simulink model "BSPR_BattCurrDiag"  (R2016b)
settings: Solver=FixedStepDiscrete  StartTime=0.0  StopTime=10.0  FixedStep=0.02  RelTol=1e-3  EnableMultiTasking=on
undefined symbols (not defined in the file): bin2dec, BSPR_cntBattCurrDiag_CW, BSPR_cntCurrChrgDiag_CW, BSPR_cntCurrStukDiag_CW, BSPR_cntPhiCurrStuk_C, BSPR_cntVehCurrStuk_C, BSPR_cofCurrChrgFlt_C, BSPR_iCurrChrgFltThres_C, BSPR_iCurrDiagAdapThres_C, BSPR_iCurrOBCDiffThres_C, BSPR_iCurrOffsDiffThres_C, BSPR_iCurrStukDiffThres_C, BSPR_PhiCurrHiDThres_C, BSPR_PhiCurrHiUThres_C, BSPR_PhiCurrLoDThres_C, BSPR_PhiCurrLoUThres_C, BSPR_tiChrgCurrDe_C, BSPR_tiChrgCurrDiagDe_C, BSPR_tiPhiCurrDe_C, BSPR_tiVehCurrDe_C, BSPR_VehCurrHiDThres_C, BSPR_VehCurrHiUThres_C, BSPR_VehCurrLoDThres_C, BSPR_VehCurrLoUThres_C
libraries: simulink x26

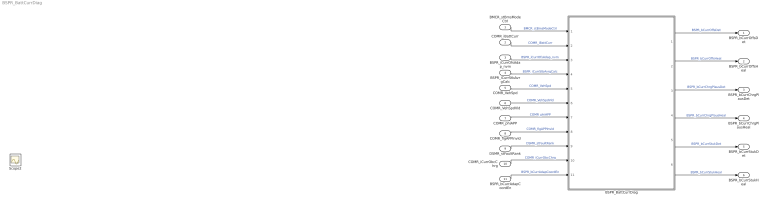
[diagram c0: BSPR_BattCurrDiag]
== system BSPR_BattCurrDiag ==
  BMCR_stBmsModeCtrl : Inport
  COMR_iBattCurr : Inport  Port=2
  BSPR_iCurrOfsAdap_nvm : Inport  Port=3
  BSPR_iCurrStbAvrgCalc : Inport  Port=4
  COMR_VehSpd : Inport  Port=5
  COMR_VehSpdVld : Inport  Port=6
  COMR_phiAPP : Inport  Port=7
  COMR_flgAPPInvld : Inport  Port=8
  DSMR_stFaultRank : Inport  Port=9
  COMR_iCurrObcChrg : Inport  Port=10
  BSPR_bCurrAdapCoordEn : Inport  Port=11
  BSPR_BattCurrDiag : Subsystem
  BSPR_bCurrOffsDet : Outport
  BSPR_bCurrOffsHeal : Outport  Port=2
  BSPR_bCurrChrgPlausDet : Outport  Port=3
  BSPR_bCurrChrgPlausHeal : Outport  Port=4
  BSPR_bCurrStukDet : Outport  Port=5
  BSPR_bCurrStukHeal : Outport  Port=6
  Scope2 : Scope
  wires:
  BMCR_stBmsModeCtrl/1 -> BSPR_BattCurrDiag/1(BMCR_stBmsModeCtrl)  "BMCR_stBmsModeCtrl"
  COMR_iBattCurr/1 -> BSPR_BattCurrDiag/2(COMR_iBattCurr)  "COMR_iBattCurr"
  BSPR_iCurrOfsAdap_nvm/1 -> BSPR_BattCurrDiag/3(BSPR_iCurrOfsAdap_nvm)  "BSPR_iCurrOfsAdap_nvm"
  COMR_iCurrObcChrg/1 -> BSPR_BattCurrDiag/10(COMR_iCurrObcChrg)  "COMR_iCurrObcChrg"
  COMR_phiAPP/1 -> BSPR_BattCurrDiag/7(COMR_phiAPP)  "COMR_phiAPP"
  COMR_VehSpd/1 -> BSPR_BattCurrDiag/5(COMR_VehSpd)  "COMR_VehSpd"
  BSPR_iCurrStbAvrgCalc/1 -> BSPR_BattCurrDiag/4(BSPR_iCurrStbAvrgCalc)  "BSPR_iCurrStbAvrgCalc"
  COMR_VehSpdVld/1 -> BSPR_BattCurrDiag/6(COMR_VehSpdVld)  "COMR_VehSpdVld"
  DSMR_stFaultRank/1 -> BSPR_BattCurrDiag/9(DSMR_stFaultRank)  "DSMR_stFaultRank"
  COMR_flgAPPInvld/1 -> BSPR_BattCurrDiag/8(COMR_flgAPPInvld)  "COMR_flgAPPInvld"
  BSPR_bCurrAdapCoordEn/1 -> BSPR_BattCurrDiag/11(BSPR_bCurrAdapCoordEn)  "BSPR_bCurrAdapCoordEn"
  BSPR_BattCurrDiag/1(BSPR_bCurrOffsDet) -> BSPR_bCurrOffsDet/1  "BSPR_bCurrOffsDet"
  BSPR_BattCurrDiag/2(BSPR_bCurrOffsHeal) -> BSPR_bCurrOffsHeal/1  "BSPR_bCurrOffsHeal"
  BSPR_BattCurrDiag/3(BSPR_bCurrChrgPlausDet) -> BSPR_bCurrChrgPlausDet/1  "BSPR_bCurrChrgPlausDet"
  BSPR_BattCurrDiag/4(BSPR_bCurrChrgPlausHeal) -> BSPR_bCurrChrgPlausHeal/1  "BSPR_bCurrChrgPlausHeal"
  BSPR_BattCurrDiag/5(BSPR_bCurrStukDet) -> BSPR_bCurrStukDet/1  "BSPR_bCurrStukDet"
  BSPR_BattCurrDiag/6(BSPR_bCurrStukHeal) -> BSPR_bCurrStukHeal/1  "BSPR_bCurrStukHeal"

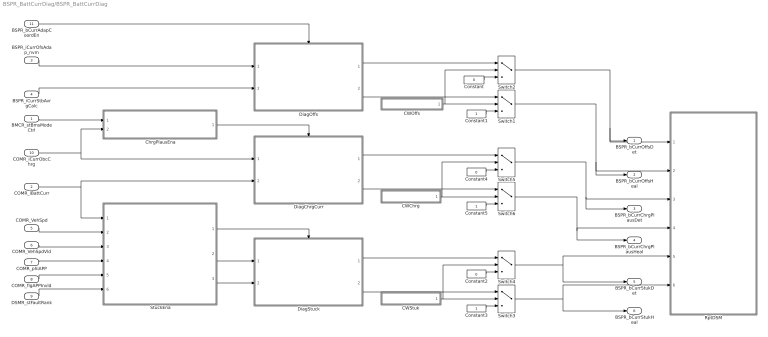
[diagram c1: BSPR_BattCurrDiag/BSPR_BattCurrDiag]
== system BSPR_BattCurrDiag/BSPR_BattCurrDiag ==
  BMCR_stBmsModeCtrl : Inport
  COMR_iBattCurr : Inport  Port=2
  BSPR_iCurrOfsAdap_nvm : Inport  Port=3
  BSPR_iCurrStbAvrgCalc : Inport  Port=4
  COMR_VehSpd : Inport  Port=5
  COMR_VehSpdVld : Inport  Port=6
  COMR_phiAPP : Inport  Port=7
  COMR_flgAPPInvld : Inport  Port=8
  DSMR_stFaultRank : Inport  Port=9
  COMR_iCurrObcChrg : Inport  Port=10
  BSPR_bCurrAdapCoordEn : Inport  Port=11
  CWChrg : Subsystem
  CWOffs : Subsystem
  CWStuk : Subsystem
  ChrgPlausEna : Subsystem  TreatAsAtomicUnit=on
  Constant : Constant  Value=0  OutDataTypeStr=boolean
  Constant1 : Constant  OutDataTypeStr=boolean
  Constant2 : Constant  Value=0  OutDataTypeStr=boolean
  Constant3 : Constant  OutDataTypeStr=boolean
  Constant4 : Constant  Value=0  OutDataTypeStr=boolean
  Constant5 : Constant  OutDataTypeStr=boolean
  DiagChrgCurr : Subsystem  TreatAsAtomicUnit=on
  DiagOffs : Subsystem
  DiagStuck : Subsystem  TreatAsAtomicUnit=on
  RptDSM : Subsystem  TreatAsAtomicUnit=on
  StuckEna : Subsystem  TreatAsAtomicUnit=on
  Switch{1..6} (6 alike) : Switch  Criteria=u2 ~= 0
  BSPR_bCurrOffsDet : Outport
  BSPR_bCurrOffsHeal : Outport  Port=2
  BSPR_bCurrChrgPlausDet : Outport  Port=3
  BSPR_bCurrChrgPlausHeal : Outport  Port=4
  BSPR_bCurrStukDet : Outport  Port=5
  BSPR_bCurrStukHeal : Outport  Port=6
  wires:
  BMCR_stBmsModeCtrl/1 -> ChrgPlausEna/1(BMCR_stBmsModeCtrl)
  BSPR_iCurrStbAvrgCalc/1 -> DiagOffs/2(BSPR_iCurrStbAvrgCalc)
  BSPR_iCurrOfsAdap_nvm/1 -> DiagOffs/1(BSPR_iCurrOfsAdap_nvm)
  StuckEna/1(BSPR_bCurrDiagStukEn) -> DiagStuck/Enable
  StuckEna/2(BSPR_iCurrMxStuk) -> DiagStuck/1(BSPR_iCurrMxStuk)
  StuckEna/3(BSPR_iCurrMnStuk) -> DiagStuck/2(BSPR_iCurrMnStuk)
  ChrgPlausEna/1(BSPR_bCurrDiagChrgPlausEn) -> DiagChrgCurr/Enable
  COMR_iCurrObcChrg/1 -> ChrgPlausEna/2(COMR_iCurrObcChrg), DiagChrgCurr/1(COMR_iCurrObcChrg)
  DSMR_stFaultRank/1 -> StuckEna/6(DSMR_stFaultRank)
  COMR_iBattCurr/1 -> StuckEna/1(COMR_iBattCurr), DiagChrgCurr/2(COMR_iBattCurr)
  COMR_flgAPPInvld/1 -> StuckEna/5(COMR_flgAPPInvld)
  COMR_phiAPP/1 -> StuckEna/4(COMR_phiAPP)
  COMR_VehSpd/1 -> StuckEna/2(COMR_VehSpd)
  COMR_VehSpdVld/1 -> StuckEna/3(COMR_VehSpdVld)
  DiagOffs/1(BSPR_bCurrOffsDet) -> Switch2/1
  Constant/1 -> Switch2/3
  CWOffs/1(~BSPR_cntBattCurrDiag_CW) -> Switch2/2, Switch1/2
  DiagOffs/2(BSPR_bCurrOffsHeal) -> Switch1/1
  Constant1/1 -> Switch1/3
  Switch2/1 -> BSPR_bCurrOffsDet/1, RptDSM/1(BSPR_bCurrOffsDet)
  Switch1/1 -> RptDSM/2(BSPR_bCurrOffsHeal), BSPR_bCurrOffsHeal/1
  CWStuk/1(BSPR_cntCurrStukDiag_CW) -> Switch4/2, Switch3/2
  DiagStuck/1(BSPR_bCurrStukDet) -> Switch4/1
  Constant2/1 -> Switch4/3
  Constant3/1 -> Switch3/3
  DiagStuck/2(BSPR_bCurrStukHeal) -> Switch3/1
  Switch4/1 -> BSPR_bCurrStukDet/1, RptDSM/5(BSPR_bCurrStukDet)
  Switch3/1 -> BSPR_bCurrStukHeal/1, RptDSM/6(BSPR_bCurrStukHeal)
  DiagChrgCurr/1(BSPR_bCurrChrgPlausDet) -> Switch5/1
  Constant4/1 -> Switch5/3
  Switch5/1 -> RptDSM/3(BSPR_bCurrChrgPlausDet), BSPR_bCurrChrgPlausDet/1
  DiagChrgCurr/2(BSPR_bCurrChrgPlausHeal) -> Switch6/1
  Constant5/1 -> Switch6/3
  CWChrg/1(BSPR_cntCurrChrgDiag_CW) -> Switch5/2, Switch6/2
  BSPR_bCurrAdapCoordEn/1 -> DiagOffs/Enable
  Switch6/1 -> BSPR_bCurrChrgPlausHeal/1, RptDSM/4(BSPR_bCurrChrgPlausHeal)

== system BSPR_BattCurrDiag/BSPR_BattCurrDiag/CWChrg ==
  Bitwise Operator : simulink/Logic and Bit Operations/Bitwise Operator  logicop=AND  UseBitMask=on  BitMask=bin2dec('00000001')  BitMaskRealWorld=Stored Integer
  Compare To Constant : simulink/Logic and Bit Operations/Compare To Constant  relop===  const=1  OutDataTypeStr=boolean
  Constant7 : Constant  Value=BSPR_cntCurrChrgDiag_CW
  BSPR_cntCurrChrgDiag_CW : Outport
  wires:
  Constant7/1 -> Bitwise Operator/1
  Bitwise Operator/1 -> Compare To Constant/1
  Compare To Constant/1 -> BSPR_cntCurrChrgDiag_CW/1

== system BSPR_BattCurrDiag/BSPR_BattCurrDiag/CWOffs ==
  Bitwise Operator : simulink/Logic and Bit Operations/Bitwise Operator  logicop=AND  UseBitMask=on  BitMask=bin2dec('00000001')  BitMaskRealWorld=Stored Integer
  Compare To Constant : simulink/Logic and Bit Operations/Compare To Constant  relop===  const=1  OutDataTypeStr=boolean
  Constant7 : Constant  Value=BSPR_cntBattCurrDiag_CW
  ~BSPR_cntBattCurrDiag_CW : Outport
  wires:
  Constant7/1 -> Bitwise Operator/1
  Bitwise Operator/1 -> Compare To Constant/1
  Compare To Constant/1 -> ~BSPR_cntBattCurrDiag_CW/1

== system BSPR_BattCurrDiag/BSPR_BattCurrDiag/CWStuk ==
  Bitwise Operator : simulink/Logic and Bit Operations/Bitwise Operator  logicop=AND  UseBitMask=on  BitMask=bin2dec('00000001')  BitMaskRealWorld=Stored Integer
  Compare To Constant : simulink/Logic and Bit Operations/Compare To Constant  relop===  const=1  OutDataTypeStr=boolean
  Constant7 : Constant  Value=BSPR_cntCurrStukDiag_CW
  BSPR_cntCurrStukDiag_CW : Outport
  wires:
  Compare To Constant/1 -> BSPR_cntCurrStukDiag_CW/1
  Bitwise Operator/1 -> Compare To Constant/1
  Constant7/1 -> Bitwise Operator/1

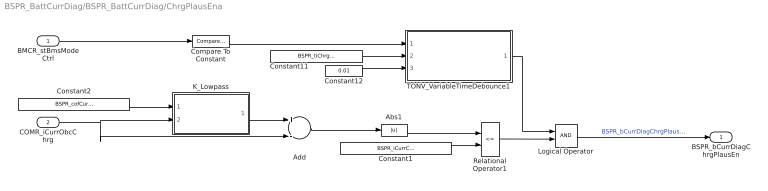
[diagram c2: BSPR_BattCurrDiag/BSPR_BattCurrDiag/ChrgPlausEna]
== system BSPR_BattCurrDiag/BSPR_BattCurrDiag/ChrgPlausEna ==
  BMCR_stBmsModeCtrl : Inport
  COMR_iCurrObcChrg : Inport  Port=2
  Abs1 : Abs
  Add : Sum  Inputs=+-
  Compare To Constant : simulink/Logic and Bit Operations/Compare To Constant  relop===  const=6  OutDataTypeStr=boolean
  Constant1 : Constant  Value=BSPR_iCurrChrgFltThres_C
  Constant11 : Constant  Value=BSPR_tiChrgCurrDe_C
  Constant12 : Constant  Value=0.01
  Constant2 : Constant  Value=BSPR_cofCurrChrgFlt_C
  K_Lowpass : Subsystem  TreatAsAtomicUnit=on  RTWFcnName=K_Lowpass  RTWFileName=SrvLib
  Logical Operator : Logic  AllPortsSameDT=off  OutDataTypeStr=boolean
  Relational Operator1 : RelationalOperator  Operator=<=  OutDataTypeStr=boolean  RndMeth=Simplest
  TONV_VariableTimeDebounce1 : Subsystem  TreatAsAtomicUnit=on  RTWFcnName=TONV_VariableTimeDebounce  RTWFileName=SrvLib
  BSPR_bCurrDiagChrgPlausEn : Outport
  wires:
  BMCR_stBmsModeCtrl/1 -> Compare To Constant/1
  Constant11/1 -> TONV_VariableTimeDebounce1/2(T)
  Constant12/1 -> TONV_VariableTimeDebounce1/3(dT)
  Compare To Constant/1 -> TONV_VariableTimeDebounce1/1(u)
  TONV_VariableTimeDebounce1/1(y) -> Logical Operator/1
  Constant1/1 -> Relational Operator1/2
  Abs1/1 -> Relational Operator1/1
  COMR_iCurrObcChrg/1 -> Add/2, K_Lowpass/2(u)
  Constant2/1 -> K_Lowpass/1(k)
  K_Lowpass/1(y) -> Add/1
  Add/1 -> Abs1/1
  Relational Operator1/1 -> Logical Operator/2
  Logical Operator/1 -> BSPR_bCurrDiagChrgPlausEn/1  "BSPR_bCurrDiagChrgPlausEn"

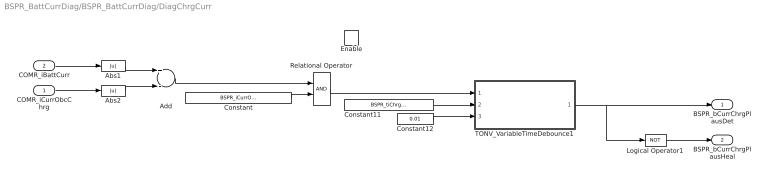
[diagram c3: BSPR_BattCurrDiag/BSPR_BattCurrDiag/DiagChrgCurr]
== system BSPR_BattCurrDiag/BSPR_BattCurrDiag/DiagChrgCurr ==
  COMR_iCurrObcChrg : Inport
  COMR_iBattCurr : Inport  Port=2
  Enable : EnablePort
  Abs1 : Abs
  Abs2 : Abs
  Add : Sum  Inputs=+-
  Constant : Constant  Value=BSPR_iCurrOBCDiffThres_C
  Constant11 : Constant  Value=BSPR_tiChrgCurrDiagDe_C
  Constant12 : Constant  Value=0.01
  Logical Operator1 : Logic  Operator=NOT  Inputs=1  AllPortsSameDT=off  OutDataTypeStr=boolean
  Relational Operator : RelationalOperator  OutDataTypeStr=boolean  RndMeth=Simplest
  TONV_VariableTimeDebounce1 : Subsystem  TreatAsAtomicUnit=on  RTWFcnName=TONV_VariableTimeDebounce  RTWFileName=SrvLib
  BSPR_bCurrChrgPlausDet : Outport
  BSPR_bCurrChrgPlausHeal : Outport  Port=2
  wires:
  COMR_iBattCurr/1 -> Abs1/1
  Constant/1 -> Relational Operator/2
  Logical Operator1/1 -> BSPR_bCurrChrgPlausHeal/1
  Constant11/1 -> TONV_VariableTimeDebounce1/2(T)
  Constant12/1 -> TONV_VariableTimeDebounce1/3(dT)
  Relational Operator/1 -> TONV_VariableTimeDebounce1/1(u)
  TONV_VariableTimeDebounce1/1(y) -> BSPR_bCurrChrgPlausDet/1, Logical Operator1/1
  Abs1/1 -> Add/1
  COMR_iCurrObcChrg/1 -> Abs2/1
  Add/1 -> Relational Operator/1
  Abs2/1 -> Add/2

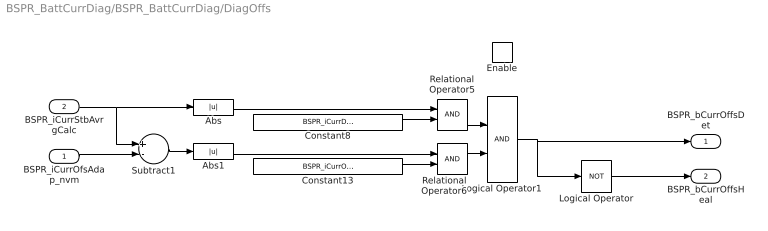
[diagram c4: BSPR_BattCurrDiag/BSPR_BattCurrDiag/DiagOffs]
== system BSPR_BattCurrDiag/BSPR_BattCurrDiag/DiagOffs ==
  BSPR_iCurrOfsAdap_nvm : Inport
  BSPR_iCurrStbAvrgCalc : Inport  Port=2
  Enable : EnablePort  StatesWhenEnabling=reset  PropagateVarSize=During execution  ZeroCross=off
  Abs : Abs
  Abs1 : Abs
  Constant13 : Constant  Value=BSPR_iCurrOffsDiffThres_C  OutDataTypeStr=single
  Constant8 : Constant  Value=BSPR_iCurrDiagAdapThres_C  OutDataTypeStr=single
  Logical Operator : Logic  Operator=NOT  Inputs=1  AllPortsSameDT=off  OutDataTypeStr=boolean
  Logical Operator1 : Logic  AllPortsSameDT=off  OutDataTypeStr=boolean
  Relational Operator5 : RelationalOperator  OutDataTypeStr=boolean  RndMeth=Simplest
  Relational Operator6 : RelationalOperator  OutDataTypeStr=boolean  RndMeth=Simplest
  Subtract1 : Sum  Inputs=+-
  BSPR_bCurrOffsDet : Outport
  BSPR_bCurrOffsHeal : Outport  Port=2
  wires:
  Constant8/1 -> Relational Operator5/2
  Constant13/1 -> Relational Operator6/2
  Logical Operator1/1 -> BSPR_bCurrOffsDet/1, Logical Operator/1
  BSPR_iCurrStbAvrgCalc/1 -> Subtract1/1, Abs/1
  Abs/1 -> Relational Operator5/1
  Subtract1/1 -> Abs1/1
  Abs1/1 -> Relational Operator6/1
  BSPR_iCurrOfsAdap_nvm/1 -> Subtract1/2
  Relational Operator5/1 -> Logical Operator1/1
  Relational Operator6/1 -> Logical Operator1/2
  Logical Operator/1 -> BSPR_bCurrOffsHeal/1

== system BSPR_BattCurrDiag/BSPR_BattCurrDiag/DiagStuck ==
  BSPR_iCurrMxStuk : Inport
  BSPR_iCurrMnStuk : Inport  Port=2
  Enable : EnablePort
  Add : Sum  Inputs=+-
  Constant : Constant  Value=BSPR_iCurrStukDiffThres_C
  Logical Operator : Logic  Operator=NOT  Inputs=1  AllPortsSameDT=off  OutDataTypeStr=boolean
  Relational Operator : RelationalOperator  Operator=<=  OutDataTypeStr=boolean  RndMeth=Simplest
  BSPR_bCurrStukDet : Outport
  BSPR_bCurrStukHeal : Outport  Port=2
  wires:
  Add/1 -> Relational Operator/1
  Constant/1 -> Relational Operator/2
  Relational Operator/1 -> Logical Operator/1, BSPR_bCurrStukDet/1
  BSPR_iCurrMxStuk/1 -> Add/1
  BSPR_iCurrMnStuk/1 -> Add/2
  Logical Operator/1 -> BSPR_bCurrStukHeal/1

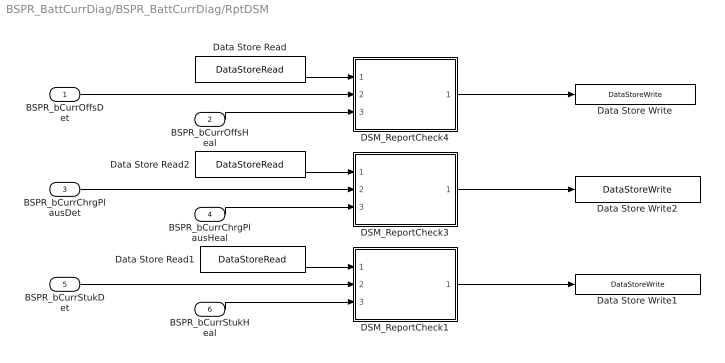
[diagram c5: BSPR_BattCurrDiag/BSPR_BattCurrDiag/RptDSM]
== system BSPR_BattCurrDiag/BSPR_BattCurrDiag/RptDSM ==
  BSPR_bCurrOffsDet : Inport
  BSPR_bCurrOffsHeal : Inport  Port=2
  BSPR_bCurrChrgPlausDet : Inport  Port=3
  BSPR_bCurrChrgPlausHeal : Inport  Port=4
  BSPR_bCurrStukDet : Inport  Port=5
  BSPR_bCurrStukHeal : Inport  Port=6
  DSM_ReportCheck1 : Subsystem  TreatAsAtomicUnit=on  RTWFcnName=DSM_ReportCheck  RTWFileName=SrvLib
  DSM_ReportCheck3 : Subsystem  TreatAsAtomicUnit=on  RTWFcnName=DSM_ReportCheck  RTWFileName=SrvLib
  DSM_ReportCheck4 : Subsystem  TreatAsAtomicUnit=on  RTWFcnName=DSM_ReportCheck  RTWFileName=SrvLib
  Data Store Read : DataStoreRead  DataStoreName=DFC_CurrOffsPlaus
  Data Store Read1 : DataStoreRead  DataStoreName=DFC_CurrStukPlaus
  Data Store Read2 : DataStoreRead  DataStoreName=DFC_CurrChrgPlaus
  Data Store Write : DataStoreWrite  DataStoreName=DFC_CurrOffsPlaus
  Data Store Write1 : DataStoreWrite  DataStoreName=DFC_CurrStukPlaus
  Data Store Write2 : DataStoreWrite  DataStoreName=DFC_CurrChrgPlaus
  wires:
  BSPR_bCurrOffsDet/1 -> DSM_ReportCheck4/2(Err)
  BSPR_bCurrOffsHeal/1 -> DSM_ReportCheck4/3(Heal)
  BSPR_bCurrStukDet/1 -> DSM_ReportCheck1/2(Err)
  BSPR_bCurrStukHeal/1 -> DSM_ReportCheck1/3(Heal)
  BSPR_bCurrChrgPlausDet/1 -> DSM_ReportCheck3/2(Err)
  BSPR_bCurrChrgPlausHeal/1 -> DSM_ReportCheck3/3(Heal)
  Data Store Read/1 -> DSM_ReportCheck4/1(Dfc_id_nv)
  DSM_ReportCheck4/1(Dfc_id) -> Data Store Write/1
  Data Store Read1/1 -> DSM_ReportCheck1/1(Dfc_id_nv)
  DSM_ReportCheck1/1(Dfc_id) -> Data Store Write1/1
  Data Store Read2/1 -> DSM_ReportCheck3/1(Dfc_id_nv)
  DSM_ReportCheck3/1(Dfc_id) -> Data Store Write2/1

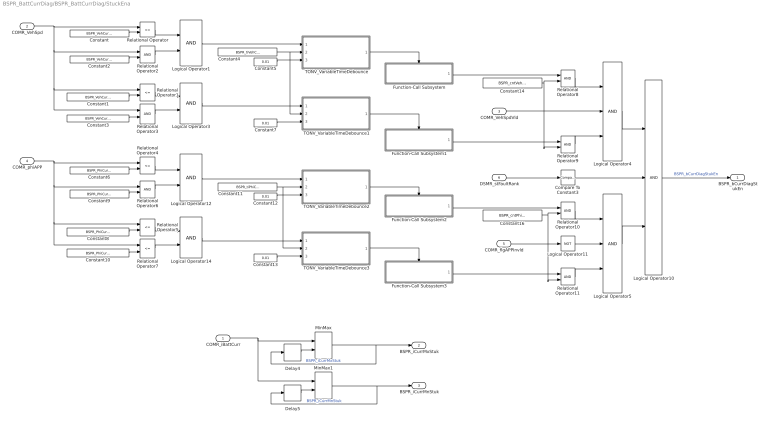
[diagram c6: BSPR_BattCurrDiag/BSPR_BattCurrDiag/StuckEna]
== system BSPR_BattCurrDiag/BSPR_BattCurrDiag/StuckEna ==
  COMR_iBattCurr : Inport
  COMR_VehSpd : Inport  Port=2
  COMR_VehSpdVld : Inport  Port=3
  COMR_phiAPP : Inport  Port=4
  COMR_flgAPPInvld : Inport  Port=5
  DSMR_stFaultRank : Inport  Port=6
  Compare To Constant3 : simulink/Logic and Bit Operations/Compare To Constant  relop=<  const=3.0  OutDataTypeStr=boolean
  Constant : Constant  Value=BSPR_VehCurrHiUThres_C
  Constant1 : Constant  Value=BSPR_VehCurrLoUThres_C
  Constant10 : Constant  Value=BSPR_PhiCurrLoDThres_C
  Constant11 : Constant  Value=BSPR_tiPhiCurrDe_C
  Constant{5,7,12..13} (4 alike) : Constant  Value=0.01
  Constant14 : Constant  Value=BSPR_cntVehCurrStuk_C
  Constant16 : Constant  Value=BSPR_cntPhiCurrStuk_C
  Constant2 : Constant  Value=BSPR_VehCurrHiDThres_C
  Constant3 : Constant  Value=BSPR_VehCurrLoDThres_C
  Constant4 : Constant  Value=BSPR_tiVehCurrDe_C
  Constant6 : Constant  Value=BSPR_PhiCurrHiUThres_C
  Constant8 : Constant  Value=BSPR_PhiCurrLoUThres_C
  Constant9 : Constant  Value=BSPR_PhiCurrHiDThres_C
  Delay4 : Delay  DelayLength=1  InitialCondition=0
  Delay5 : Delay  DelayLength=1  InitialCondition=0
  Function-Call Subsystem : Subsystem  TreatAsAtomicUnit=on
  Function-Call Subsystem1 : Subsystem  TreatAsAtomicUnit=on
  Function-Call Subsystem2 : Subsystem  TreatAsAtomicUnit=on
  Function-Call Subsystem3 : Subsystem  TreatAsAtomicUnit=on
  Logical Operator{1,3,12,14} (4 alike) : Logic  AllPortsSameDT=off  OutDataTypeStr=boolean
  Logical Operator10 : Logic  Inputs=3  AllPortsSameDT=off  OutDataTypeStr=boolean
  Logical Operator11 : Logic  Operator=NOT  Inputs=1  AllPortsSameDT=off  OutDataTypeStr=boolean
  Logical Operator4 : Logic  Inputs=3  AllPortsSameDT=off  OutDataTypeStr=boolean
  Logical Operator5 : Logic  Inputs=3  AllPortsSameDT=off  OutDataTypeStr=boolean
  MinMax : MinMax  Function=max  Inputs=2
  MinMax1 : MinMax  Inputs=2
  Relational Operator{,1,4..5,7} (5 alike) : RelationalOperator  Operator=<=  OutDataTypeStr=boolean  RndMeth=Simplest
  Relational Operator{2..3,6,8..11} (7 alike) : RelationalOperator  OutDataTypeStr=boolean  RndMeth=Simplest
  TONV_VariableTimeDebounce : Subsystem  TreatAsAtomicUnit=on  RTWFcnName=TONV_VariableTimeDebounce  RTWFileName=SrvLib
  TONV_VariableTimeDebounce1 : Subsystem  TreatAsAtomicUnit=on  RTWFcnName=TONV_VariableTimeDebounce  RTWFileName=SrvLib
  TONV_VariableTimeDebounce2 : Subsystem  TreatAsAtomicUnit=on  RTWFcnName=TONV_VariableTimeDebounce  RTWFileName=SrvLib
  TONV_VariableTimeDebounce3 : Subsystem  TreatAsAtomicUnit=on  RTWFcnName=TONV_VariableTimeDebounce  RTWFileName=SrvLib
  BSPR_bCurrDiagStukEn : Outport
  BSPR_iCurrMxStuk : Outport  Port=2
  BSPR_iCurrMnStuk : Outport  Port=3
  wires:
  COMR_VehSpd/1 -> Relational Operator/1, Relational Operator2/1, Relational Operator1/1, Relational Operator3/1
  DSMR_stFaultRank/1 -> Compare To Constant3/1
  Logical Operator4/1 -> Logical Operator10/1
  Logical Operator10/1 -> BSPR_bCurrDiagStukEn/1  "BSPR_bCurrDiagStukEn"
  Delay4/1 -> MinMax/2
  COMR_iBattCurr/1 -> MinMax1/1, MinMax/1
  MinMax/1 -> BSPR_iCurrMxStuk/1, Delay4/1  "BSPR_iCurrMxStuk"
  Delay5/1 -> MinMax1/2
  MinMax1/1 -> BSPR_iCurrMnStuk/1, Delay5/1  "BSPR_iCurrMnStuk"
  COMR_flgAPPInvld/1 -> Logical Operator11/1
  Constant/1 -> Relational Operator/2
  Constant2/1 -> Relational Operator2/2
  Constant1/1 -> Relational Operator1/2
  Relational Operator1/1 -> Logical Operator3/1
  Relational Operator3/1 -> Logical Operator3/2
  Constant3/1 -> Relational Operator3/2
  Relational Operator/1 -> Logical Operator1/1
  Relational Operator2/1 -> Logical Operator1/2
  Logical Operator1/1 -> TONV_VariableTimeDebounce/1(u)
  Constant4/1 -> TONV_VariableTimeDebounce1/2(T), TONV_VariableTimeDebounce/2(T)
  Constant5/1 -> TONV_VariableTimeDebounce/3(dT)
  TONV_VariableTimeDebounce/1(y) -> Function-Call Subsystem/Trigger
  Logical Operator3/1 -> TONV_VariableTimeDebounce1/1(u)
  Constant7/1 -> TONV_VariableTimeDebounce1/3(dT)
  COMR_phiAPP/1 -> Relational Operator7/1, Relational Operator5/1, Relational Operator6/1, Relational Operator4/1
  Constant6/1 -> Relational Operator4/2
  Constant9/1 -> Relational Operator6/2
  Constant8/1 -> Relational Operator5/2
  Relational Operator5/1 -> Logical Operator14/1
  Relational Operator7/1 -> Logical Operator14/2
  Constant10/1 -> Relational Operator7/2
  Relational Operator4/1 -> Logical Operator12/1
  Relational Operator6/1 -> Logical Operator12/2
  Logical Operator12/1 -> TONV_VariableTimeDebounce2/1(u)
  Constant11/1 -> TONV_VariableTimeDebounce3/2(T), TONV_VariableTimeDebounce2/2(T)
  Constant12/1 -> TONV_VariableTimeDebounce2/3(dT)
  Logical Operator14/1 -> TONV_VariableTimeDebounce3/1(u)
  Constant13/1 -> TONV_VariableTimeDebounce3/3(dT)
  COMR_VehSpdVld/1 -> Logical Operator4/2
  Logical Operator11/1 -> Logical Operator5/2
  Logical Operator5/1 -> Logical Operator10/3
  Compare To Constant3/1 -> Logical Operator10/2
  Relational Operator8/1 -> Logical Operator4/1
  Function-Call Subsystem/1(BSPR_cntCurrVehStukUp) -> Relational Operator8/1
  Constant14/1 -> Relational Operator9/2, Relational Operator8/2
  Relational Operator9/1 -> Logical Operator4/3
  Function-Call Subsystem1/1(BSPR_cntCurrVehStukLo) -> Relational Operator9/1
  Constant16/1 -> Relational Operator11/2, Relational Operator10/2
  Relational Operator10/1 -> Logical Operator5/1
  Function-Call Subsystem2/1(BSPR_cntCurrPedStukUp) -> Relational Operator10/1
  Relational Operator11/1 -> Logical Operator5/3
  Function-Call Subsystem3/1(BSPR_cntCurrPedStukLo) -> Relational Operator11/1
  TONV_VariableTimeDebounce1/1(y) -> Function-Call Subsystem1/Trigger
  TONV_VariableTimeDebounce2/1(y) -> Function-Call Subsystem2/Trigger
  TONV_VariableTimeDebounce3/1(y) -> Function-Call Subsystem3/Trigger

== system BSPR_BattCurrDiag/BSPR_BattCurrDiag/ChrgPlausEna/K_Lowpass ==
  k : Inport
  u : Inport  Port=2
  Add : Sum
  Constant2 : Constant  Value=0
  Delay : Delay  DelayLength=1  InitialCondition=1
  Product : Product
  Subtract : Sum  Inputs=+-
  Switch1 : Switch  Criteria=u2 > Threshold
  Unit Delay : UnitDelay  SampleTime=-1
  y : Outport
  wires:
  u/1 -> Subtract/1, Switch1/1
  Switch1/1 -> Unit Delay/1, y/1
  Delay/1 -> Switch1/2
  Add/1 -> Switch1/3
  Subtract/1 -> Product/2
  Unit Delay/1 -> Add/2, Subtract/2
  Constant2/1 -> Delay/1
  Product/1 -> Add/1
  k/1 -> Product/1

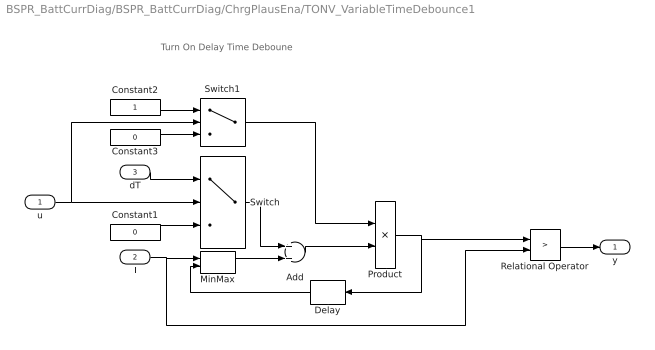
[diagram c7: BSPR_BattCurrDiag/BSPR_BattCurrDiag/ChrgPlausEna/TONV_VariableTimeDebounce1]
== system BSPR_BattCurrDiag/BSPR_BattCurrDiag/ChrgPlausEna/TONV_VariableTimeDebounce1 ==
  note: Turn On Delay Time Deboune
  u : Inport
  T : Inport  Port=2
  dT : Inport  Port=3
  Add : Sum
  Constant1 : Constant  Value=0  OutDataTypeStr=single
  Constant2 : Constant  OutDataTypeStr=uint8
  Constant3 : Constant  Value=0  OutDataTypeStr=uint8
  Delay : Delay  DelayLength=1  InitialCondition=0
  MinMax : MinMax  Inputs=2
  Product : Product  OutMin=[0]  OutMax=[65535]  OutDataTypeStr=single
  Relational Operator : RelationalOperator  Operator=>  OutDataTypeStr=boolean  RndMeth=Simplest
  Switch : Switch  Criteria=u2 ~= 0
  Switch1 : Switch  Criteria=u2 ~= 0
  y : Outport
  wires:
  MinMax/1 -> Add/2
  T/1 -> Relational Operator/2, MinMax/1
  Relational Operator/1 -> y/1
  Delay/1 -> MinMax/2
  Switch/1 -> Add/1
  Product/1 -> Delay/1, Relational Operator/1
  Add/1 -> Product/2
  Constant1/1 -> Switch/3
  dT/1 -> Switch/1
  u/1 -> Switch/2, Switch1/2
  Constant2/1 -> Switch1/1
  Constant3/1 -> Switch1/3
  Switch1/1 -> Product/1

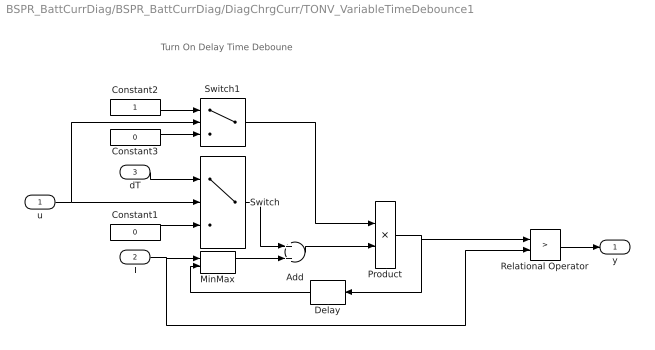
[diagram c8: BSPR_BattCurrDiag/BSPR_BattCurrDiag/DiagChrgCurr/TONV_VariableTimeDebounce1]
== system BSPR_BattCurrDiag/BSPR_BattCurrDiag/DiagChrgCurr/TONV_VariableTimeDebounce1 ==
  note: Turn On Delay Time Deboune
  u : Inport
  T : Inport  Port=2
  dT : Inport  Port=3
  Add : Sum
  Constant1 : Constant  Value=0  OutDataTypeStr=single
  Constant2 : Constant  OutDataTypeStr=uint8
  Constant3 : Constant  Value=0  OutDataTypeStr=uint8
  Delay : Delay  DelayLength=1  InitialCondition=0
  MinMax : MinMax  Inputs=2
  Product : Product  OutMin=[0]  OutMax=[65535]  OutDataTypeStr=single
  Relational Operator : RelationalOperator  Operator=>  OutDataTypeStr=boolean  RndMeth=Simplest
  Switch : Switch  Criteria=u2 ~= 0
  Switch1 : Switch  Criteria=u2 ~= 0
  y : Outport
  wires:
  MinMax/1 -> Add/2
  T/1 -> Relational Operator/2, MinMax/1
  Relational Operator/1 -> y/1
  Delay/1 -> MinMax/2
  Switch/1 -> Add/1
  Product/1 -> Delay/1, Relational Operator/1
  Add/1 -> Product/2
  Constant1/1 -> Switch/3
  dT/1 -> Switch/1
  u/1 -> Switch/2, Switch1/2
  Constant2/1 -> Switch1/1
  Constant3/1 -> Switch1/3
  Switch1/1 -> Product/1

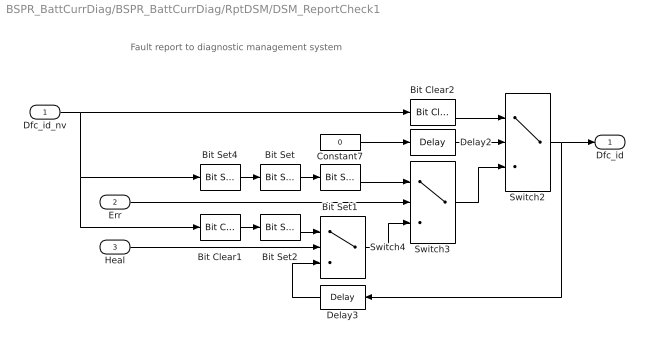
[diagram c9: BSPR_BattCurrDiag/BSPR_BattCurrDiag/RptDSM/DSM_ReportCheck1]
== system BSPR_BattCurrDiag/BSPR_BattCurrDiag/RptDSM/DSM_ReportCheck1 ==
  note: Fault report to diagnostic management system
  Dfc_id_nv : Inport  OutDataTypeStr=uint8
  Err : Inport  Port=2
  Heal : Inport  Port=3
  Bit Clear1 : simulink/Logic and Bit Operations/Bit Clear  iBit=4
  Bit Clear2 : simulink/Logic and Bit Operations/Bit Clear  iBit=3
  Bit Set : simulink/Logic and Bit Operations/Bit Set  iBit=4
  Bit Set1 : simulink/Logic and Bit Operations/Bit Set  iBit=3
  Bit Set2 : simulink/Logic and Bit Operations/Bit Set  iBit=3
  Bit Set4 : simulink/Logic and Bit Operations/Bit Set  iBit=7
  Constant7 : Constant  Value=0  OutDataTypeStr=boolean
  Delay2 : Delay  DelayLength=1  InitialCondition=1
  Delay3 : Delay  DelayLength=1  InitialCondition=0
  Switch2 : Switch  Criteria=u2 ~= 0
  Switch3 : Switch  Criteria=u2 ~= 0
  Switch4 : Switch  Criteria=u2 ~= 0
  Dfc_id : Outport  OutDataTypeStr=uint8
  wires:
  Heal/1 -> Switch4/2
  Delay3/1 -> Switch4/3
  Bit Clear1/1 -> Bit Set2/1
  Bit Set2/1 -> Switch4/1
  Err/1 -> Switch3/2
  Switch4/1 -> Switch3/3
  Bit Set/1 -> Bit Set1/1
  Bit Set1/1 -> Switch3/1
  Switch2/1 -> Dfc_id/1, Delay3/1
  Bit Clear2/1 -> Switch2/1
  Switch3/1 -> Switch2/3
  Delay2/1 -> Switch2/2
  Constant7/1 -> Delay2/1
  Bit Set4/1 -> Bit Set/1
  Dfc_id_nv/1 -> Bit Clear1/1, Bit Set4/1, Bit Clear2/1

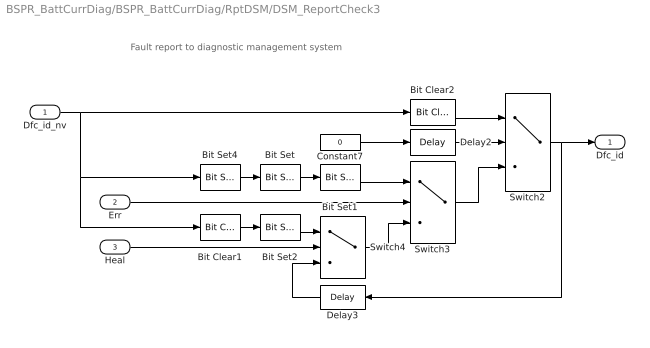
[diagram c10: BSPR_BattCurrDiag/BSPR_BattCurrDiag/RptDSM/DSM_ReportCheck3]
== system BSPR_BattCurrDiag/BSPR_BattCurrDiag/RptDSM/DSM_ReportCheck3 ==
  note: Fault report to diagnostic management system
  Dfc_id_nv : Inport  OutDataTypeStr=uint8
  Err : Inport  Port=2
  Heal : Inport  Port=3
  Bit Clear1 : simulink/Logic and Bit Operations/Bit Clear  iBit=4
  Bit Clear2 : simulink/Logic and Bit Operations/Bit Clear  iBit=3
  Bit Set : simulink/Logic and Bit Operations/Bit Set  iBit=4
  Bit Set1 : simulink/Logic and Bit Operations/Bit Set  iBit=3
  Bit Set2 : simulink/Logic and Bit Operations/Bit Set  iBit=3
  Bit Set4 : simulink/Logic and Bit Operations/Bit Set  iBit=7
  Constant7 : Constant  Value=0  OutDataTypeStr=boolean
  Delay2 : Delay  DelayLength=1  InitialCondition=1
  Delay3 : Delay  DelayLength=1  InitialCondition=0
  Switch2 : Switch  Criteria=u2 ~= 0
  Switch3 : Switch  Criteria=u2 ~= 0
  Switch4 : Switch  Criteria=u2 ~= 0
  Dfc_id : Outport  OutDataTypeStr=uint8
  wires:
  Dfc_id_nv/1 -> Bit Clear2/1, Bit Set4/1, Bit Clear1/1
  Bit Set4/1 -> Bit Set/1
  Constant7/1 -> Delay2/1
  Delay2/1 -> Switch2/2
  Switch3/1 -> Switch2/3
  Bit Clear2/1 -> Switch2/1
  Switch2/1 -> Delay3/1, Dfc_id/1
  Bit Set1/1 -> Switch3/1
  Bit Set/1 -> Bit Set1/1
  Switch4/1 -> Switch3/3
  Err/1 -> Switch3/2
  Bit Set2/1 -> Switch4/1
  Bit Clear1/1 -> Bit Set2/1
  Delay3/1 -> Switch4/3
  Heal/1 -> Switch4/2

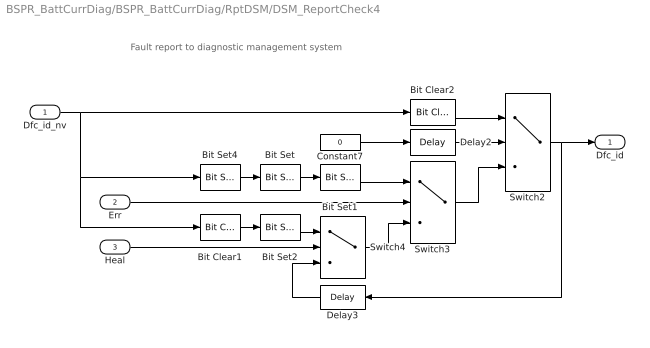
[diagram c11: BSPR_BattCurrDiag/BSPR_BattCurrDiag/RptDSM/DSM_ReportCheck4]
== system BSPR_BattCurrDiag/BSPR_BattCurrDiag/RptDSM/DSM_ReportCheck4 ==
  note: Fault report to diagnostic management system
  Dfc_id_nv : Inport  OutDataTypeStr=uint8
  Err : Inport  Port=2
  Heal : Inport  Port=3
  Bit Clear1 : simulink/Logic and Bit Operations/Bit Clear  iBit=4
  Bit Clear2 : simulink/Logic and Bit Operations/Bit Clear  iBit=3
  Bit Set : simulink/Logic and Bit Operations/Bit Set  iBit=4
  Bit Set1 : simulink/Logic and Bit Operations/Bit Set  iBit=3
  Bit Set2 : simulink/Logic and Bit Operations/Bit Set  iBit=3
  Bit Set4 : simulink/Logic and Bit Operations/Bit Set  iBit=7
  Constant7 : Constant  Value=0  OutDataTypeStr=boolean
  Delay2 : Delay  DelayLength=1  InitialCondition=1
  Delay3 : Delay  DelayLength=1  InitialCondition=0
  Switch2 : Switch  Criteria=u2 ~= 0
  Switch3 : Switch  Criteria=u2 ~= 0
  Switch4 : Switch  Criteria=u2 ~= 0
  Dfc_id : Outport  OutDataTypeStr=uint8
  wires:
  Heal/1 -> Switch4/2
  Delay3/1 -> Switch4/3
  Bit Clear1/1 -> Bit Set2/1
  Bit Set2/1 -> Switch4/1
  Err/1 -> Switch3/2
  Switch4/1 -> Switch3/3
  Bit Set/1 -> Bit Set1/1
  Bit Set1/1 -> Switch3/1
  Switch2/1 -> Dfc_id/1, Delay3/1
  Bit Clear2/1 -> Switch2/1
  Switch3/1 -> Switch2/3
  Delay2/1 -> Switch2/2
  Constant7/1 -> Delay2/1
  Bit Set4/1 -> Bit Set/1
  Dfc_id_nv/1 -> Bit Clear1/1, Bit Set4/1, Bit Clear2/1

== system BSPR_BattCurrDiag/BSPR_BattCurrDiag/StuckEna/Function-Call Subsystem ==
  function : TriggerPort  VariantControl=Variant
  Add : Sum
  Constant2 : Constant  Value=uint8(1)
  Delay : Delay  DelayLength=1  InitialCondition=0
  BSPR_cntCurrVehStukUp : Outport
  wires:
  Add/1 -> Delay/1, BSPR_cntCurrVehStukUp/1  "BSPR_cntCurrVehStukUp"
  Constant2/1 -> Add/1
  Delay/1 -> Add/2

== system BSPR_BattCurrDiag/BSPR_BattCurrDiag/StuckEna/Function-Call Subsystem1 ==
  function : TriggerPort  VariantControl=Variant
  Add : Sum
  Constant1 : Constant  Value=uint8(1)
  Delay : Delay  DelayLength=1  InitialCondition=0
  BSPR_cntCurrVehStukLo : Outport
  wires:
  Constant1/1 -> Add/1
  Add/1 -> BSPR_cntCurrVehStukLo/1, Delay/1  "BSPR_cntCurrVehStukLo"
  Delay/1 -> Add/2

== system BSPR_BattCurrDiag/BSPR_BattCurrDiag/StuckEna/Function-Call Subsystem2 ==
  function : TriggerPort  VariantControl=Variant
  Add : Sum
  Constant : Constant  Value=uint8(1)
  Delay : Delay  DelayLength=1  InitialCondition=0
  BSPR_cntCurrPedStukUp : Outport
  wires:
  Add/1 -> Delay/1, BSPR_cntCurrPedStukUp/1  "BSPR_cntCurrPedStukUp"
  Constant/1 -> Add/1
  Delay/1 -> Add/2

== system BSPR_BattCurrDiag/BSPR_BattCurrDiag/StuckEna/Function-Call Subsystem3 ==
  function : TriggerPort  VariantControl=Variant
  Add : Sum
  Constant1 : Constant  Value=uint8(1)
  Delay : Delay  DelayLength=1  InitialCondition=0
  BSPR_cntCurrPedStukLo : Outport
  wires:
  Constant1/1 -> Add/1
  Add/1 -> BSPR_cntCurrPedStukLo/1, Delay/1  "BSPR_cntCurrPedStukLo"
  Delay/1 -> Add/2

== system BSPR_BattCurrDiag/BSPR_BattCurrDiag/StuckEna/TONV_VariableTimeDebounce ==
  note: Turn On Delay Time Deboune
  u : Inport
  T : Inport  Port=2
  dT : Inport  Port=3
  Add : Sum
  Constant1 : Constant  Value=0  OutDataTypeStr=single
  Constant2 : Constant  OutDataTypeStr=uint8
  Constant3 : Constant  Value=0  OutDataTypeStr=uint8
  Delay : Delay  DelayLength=1  InitialCondition=0
  MinMax : MinMax  Inputs=2
  Product : Product  OutMin=[0]  OutMax=[65535]  OutDataTypeStr=single
  Relational Operator : RelationalOperator  Operator=>  OutDataTypeStr=boolean  RndMeth=Simplest
  Switch : Switch  Criteria=u2 ~= 0
  Switch1 : Switch  Criteria=u2 ~= 0
  y : Outport
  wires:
  Switch1/1 -> Product/1
  Constant3/1 -> Switch1/3
  Constant2/1 -> Switch1/1
  u/1 -> Switch1/2, Switch/2
  dT/1 -> Switch/1
  Constant1/1 -> Switch/3
  Add/1 -> Product/2
  Product/1 -> Relational Operator/1, Delay/1
  Switch/1 -> Add/1
  Delay/1 -> MinMax/2
  Relational Operator/1 -> y/1
  T/1 -> MinMax/1, Relational Operator/2
  MinMax/1 -> Add/2

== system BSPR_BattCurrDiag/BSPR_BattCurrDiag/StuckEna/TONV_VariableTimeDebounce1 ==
  note: Turn On Delay Time Deboune
  u : Inport
  T : Inport  Port=2
  dT : Inport  Port=3
  Add : Sum
  Constant1 : Constant  Value=0  OutDataTypeStr=single
  Constant2 : Constant  OutDataTypeStr=uint8
  Constant3 : Constant  Value=0  OutDataTypeStr=uint8
  Delay : Delay  DelayLength=1  InitialCondition=0
  MinMax : MinMax  Inputs=2
  Product : Product  OutMin=[0]  OutMax=[65535]  OutDataTypeStr=single
  Relational Operator : RelationalOperator  Operator=>  OutDataTypeStr=boolean  RndMeth=Simplest
  Switch : Switch  Criteria=u2 ~= 0
  Switch1 : Switch  Criteria=u2 ~= 0
  y : Outport
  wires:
  MinMax/1 -> Add/2
  T/1 -> Relational Operator/2, MinMax/1
  Relational Operator/1 -> y/1
  Delay/1 -> MinMax/2
  Switch/1 -> Add/1
  Product/1 -> Delay/1, Relational Operator/1
  Add/1 -> Product/2
  Constant1/1 -> Switch/3
  dT/1 -> Switch/1
  u/1 -> Switch/2, Switch1/2
  Constant2/1 -> Switch1/1
  Constant3/1 -> Switch1/3
  Switch1/1 -> Product/1

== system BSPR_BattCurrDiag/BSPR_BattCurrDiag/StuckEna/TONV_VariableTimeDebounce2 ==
  note: Turn On Delay Time Deboune
  u : Inport
  T : Inport  Port=2
  dT : Inport  Port=3
  Add : Sum
  Constant1 : Constant  Value=0  OutDataTypeStr=single
  Constant2 : Constant  OutDataTypeStr=uint8
  Constant3 : Constant  Value=0  OutDataTypeStr=uint8
  Delay : Delay  DelayLength=1  InitialCondition=0
  MinMax : MinMax  Inputs=2
  Product : Product  OutMin=[0]  OutMax=[65535]  OutDataTypeStr=single
  Relational Operator : RelationalOperator  Operator=>  OutDataTypeStr=boolean  RndMeth=Simplest
  Switch : Switch  Criteria=u2 ~= 0
  Switch1 : Switch  Criteria=u2 ~= 0
  y : Outport
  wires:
  Switch1/1 -> Product/1
  Constant3/1 -> Switch1/3
  Constant2/1 -> Switch1/1
  u/1 -> Switch1/2, Switch/2
  dT/1 -> Switch/1
  Constant1/1 -> Switch/3
  Add/1 -> Product/2
  Product/1 -> Relational Operator/1, Delay/1
  Switch/1 -> Add/1
  Delay/1 -> MinMax/2
  Relational Operator/1 -> y/1
  T/1 -> MinMax/1, Relational Operator/2
  MinMax/1 -> Add/2

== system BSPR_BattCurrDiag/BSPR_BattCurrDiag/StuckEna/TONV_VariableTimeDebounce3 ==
  note: Turn On Delay Time Deboune
  u : Inport
  T : Inport  Port=2
  dT : Inport  Port=3
  Add : Sum
  Constant1 : Constant  Value=0  OutDataTypeStr=single
  Constant2 : Constant  OutDataTypeStr=uint8
  Constant3 : Constant  Value=0  OutDataTypeStr=uint8
  Delay : Delay  DelayLength=1  InitialCondition=0
  MinMax : MinMax  Inputs=2
  Product : Product  OutMin=[0]  OutMax=[65535]  OutDataTypeStr=single
  Relational Operator : RelationalOperator  Operator=>  OutDataTypeStr=boolean  RndMeth=Simplest
  Switch : Switch  Criteria=u2 ~= 0
  Switch1 : Switch  Criteria=u2 ~= 0
  y : Outport
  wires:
  MinMax/1 -> Add/2
  T/1 -> Relational Operator/2, MinMax/1
  Relational Operator/1 -> y/1
  Delay/1 -> MinMax/2
  Switch/1 -> Add/1
  Product/1 -> Delay/1, Relational Operator/1
  Add/1 -> Product/2
  Constant1/1 -> Switch/3
  dT/1 -> Switch/1
  u/1 -> Switch/2, Switch1/2
  Constant2/1 -> Switch1/1
  Constant3/1 -> Switch1/3
  Switch1/1 -> Product/1
